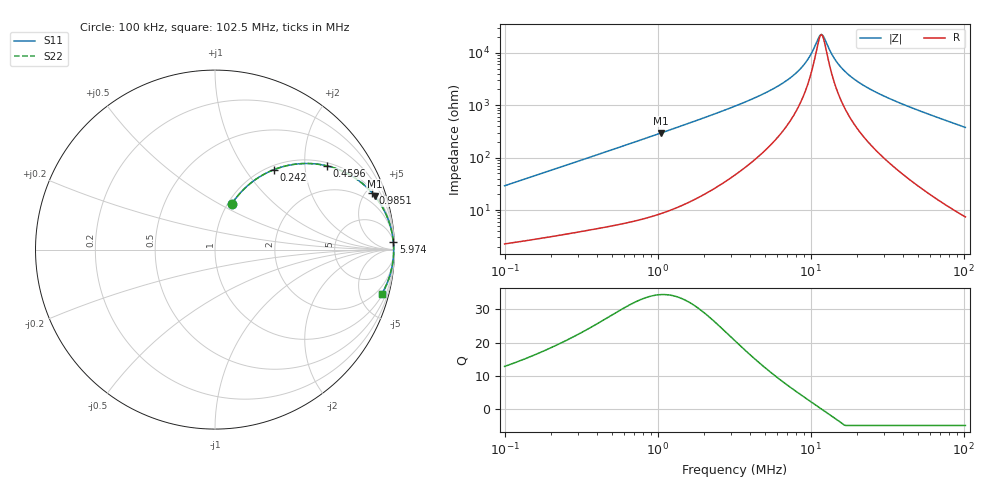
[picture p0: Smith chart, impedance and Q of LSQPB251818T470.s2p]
! LSQPB251818T470  S-PARAMETER MODEL  ( General Type )
! Model Generated by TAIYO YUDEN Corporation (http://www.ty-top.com)
! Version 2.0
! TAIYO YUDEN Control No. 100810NG19SB-FKC
! Copyright(c) 2009 TAIYO YUDEN CO.,LTD. All Rights Reserved.
! Product Description (link to TY-COMPAS)
! https://ds.yuden.co.jp/TYCOMPAS/or/detail?pn=LSQPB251818T470K&u=M
! Products Name : Inductors
! Characteristics :
!  Inductance : 47 uH , SRF(min) : 6.5 MHz , DC Resistance(max) : 1.885 Ohm
!  Rated Current : Saturation :410 mA , Temp Rise : 300 mA (40 degC)
!  Case Size : 2.5 x 1.8 / 0.098 x 0.071 [mm/inch] , Thickness : 1.8 / 0.071 [mm/inch]
!  (Conditions: Temperature = 25 degC , DC Bias Current/Voltage = 0A / 0V)
! External Node Assignments :
!  1  o---GGG---o  2
! GND o---------o GND
! Frequency Range : 0.1MHz  -  102.47202MHz  [ 402 STEP ]
# MHz S RI R 50
! Freq[MHz].  S11 Real  S11 Imag  S21 Real  S21 Imag  S12 Real  S12 Imag  S22 Real  S22 Imag
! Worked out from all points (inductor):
!   401 points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, 100 kHz to 102.5 MHz, reference 50 ohm
!   read as one part in series: L = 45.8 uH near 103.5 kHz
!   highest Q = 34.5 at 1.056 MHz (marker M1), where L = 44.7 uH
!   self-resonance near 11.54 MHz
!   S11 on the Smith chart (normalised r, x): 100 kHz: 1.05, +0.58; 242 kHz: 1.07, +1.38; 459.6 kHz: 1.09, +2.58; 985.1 kHz: 1.16, +5.53; 5.974 MHz: 6, +44; 102.5 MHz: 1.15, -7.55
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0.1  0.0948 0.2565  0.9052 -0.2565  0.9052 -0.2565  0.0948 0.2565
0.156924  0.1834 0.3575  0.8166 -0.3575  0.8166 -0.3575  0.1834 0.3575
0.242021  0.3294 0.4459  0.6706 -0.4459  0.6706 -0.4459  0.3294 0.4459
0.319357  0.4515 0.4765  0.5485 -0.4765  0.5485 -0.4765  0.4515 0.4765
0.45955  0.6215 0.467  0.3785 -0.467  0.3785 -0.467  0.6215 0.467
0.672847  0.7737 0.4029  0.2263 -0.4029  0.2263 -0.4029  0.7737 0.4029
0.985144  0.8774 0.3137  0.1226 -0.3137  0.1226 -0.3137  0.8774 0.3137
1.019889  0.8845 0.3055  0.1155 -0.3055  0.1155 -0.3055  0.8845 0.3055
1.055859  0.8911 0.2973  0.1089 -0.2973  0.1089 -0.2973  0.8911 0.2973
1.715332  0.954 0.1942  0.046 -0.1942  0.046 -0.1942  0.954 0.1942
3.257086  0.9849 0.0998  0.0151 -0.0998  0.0151 -0.0998  0.9849 0.0998
5.973889  0.9934 0.0441  0.00656 -0.0441  0.00656 -0.0441  0.9934 0.0441
8.303494  0.995 0.0214  0.00497 -0.0214  0.00497 -0.0214  0.995 0.0214
9.374465  0.9953 0.0138  0.00468 -0.0138  0.00468 -0.0138  0.9953 0.0138
10.22302  0.9955 0.00842  0.00454 -0.00842  0.00454 -0.00842  0.9955 0.00842
11.34327  0.9955 0.00208  0.00446 -0.00208  0.00446 -0.00208  0.9955 0.00208
11.94862  0.9956 -0.00108  0.00445 0.00108  0.00445 0.00108  0.9956 -0.00108
14.20963  0.9954 -0.0117  0.00456 0.0117  0.00456 0.0117  0.9954 -0.0117
16.89849  0.9951 -0.0226  0.00492 0.0226  0.00492 0.0226  0.9951 -0.0226
22.29832  0.9939 -0.0417  0.00612 0.0417  0.00612 0.0417  0.9939 -0.0417
32.64791  0.9902 -0.0733  0.00979 0.0733  0.00979 0.0733  0.9902 -0.0733
102.472  0.9302 -0.2451  0.0698 0.2451  0.0698 0.2451  0.9302 -0.2451
